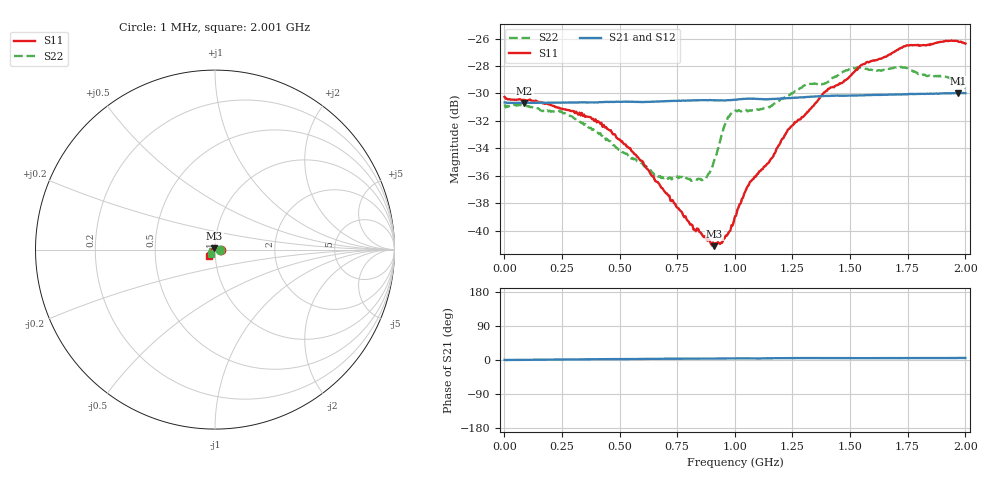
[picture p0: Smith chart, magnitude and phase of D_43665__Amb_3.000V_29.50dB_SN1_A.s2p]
! device id: 43665_
! dir: \\malibu\benchdata\1_engineers\tn_data\43665_75ohm\new\sparar\43665_\amb\3p000v\29p50db
! Serial: 1
! Insertion: A
! Temp: Amb
! VDD: 3.000V
! Attenuation Step: 29.50dB
! IDD: 1.450117e+00mA
! FILE NAME
! DATE 03-27-2009 08:40:42
! CORRECTED  DATA
#  Hz  S  RI  R  75
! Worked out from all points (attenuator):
!   401 points, 1 MHz to 2.001 GHz, reference 75 ohm
!   highest |S21| = -29.97 dB at 1.971 GHz (marker M1); lowest = -30.7 dB at 86 MHz (marker M2)
!   lowest |S11| = -41.1 dB at 911 MHz (marker M3), VSWR 1.02, Z = 74.4 + j1.16 ohm
!   |S11| at or under -10 dB: start of sweep to end of sweep
!   |S22| runs from -36.4 to -28.1 dB; largest |S21 - S12| = 0.00043
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1000000  0.0307 -0.000332  0.0293 0.000221  0.0293 -0.000151  0.0288 -0.000389
8.6e7  0.0299 0.00228  0.0292 0.000245  0.0292 0.000214  0.0283 0.0047
2.41e8  0.0272 0.00616  0.0293 0.000641  0.0293 0.000677  0.0245 0.0117
3.36e8  0.0256 0.00816  0.0293 0.000856  0.0293 0.000866  0.0195 0.0151
4.71e8  0.0197 0.0107  0.0294 0.0012  0.0295 0.00124  0.0118 0.0168
5.91e8  0.014 0.0113  0.0294 0.00139  0.0294 0.00141  0.0033 0.0174
6.71e8  0.00998 0.011  0.0295 0.00168  0.0295 0.00169  -0.00116 0.0157
8.66e8  -0.000993 0.00942  0.0298 0.00188  0.0298 0.00198  -0.0137 0.00713
9.11e8  -0.00409 0.00778  0.0298 0.00192  0.0298 0.00203  -0.0177 0.00389
9.61e8  -0.00677 0.00682  0.0298 0.00213  0.0298 0.0022  -0.0245 0.00322
1.001e9  -0.00933 0.00634  0.0299 0.00234  0.0299 0.0024  -0.027 0.00448
1.066e9  -0.0144 0.00441  0.0302 0.00226  0.0302 0.00234  -0.0274 0.00137
1.156e9  -0.0182 0.00122  0.0301 0.00245  0.0301 0.00256  -0.0283 -0.0028
1.236e9  -0.0234 -0.00229  0.0303 0.00262  0.0304 0.00277  -0.0302 -0.008
1.336e9  -0.0274 -0.00715  0.0307 0.00274  0.0307 0.00283  -0.0317 -0.013
1.396e9  -0.0304 -0.0108  0.0309 0.00265  0.0309 0.0028  -0.0302 -0.0167
1.471e9  -0.0317 -0.0144  0.0309 0.00262  0.031 0.00273  -0.0324 -0.0199
1.546e9  -0.0354 -0.0185  0.031 0.00268  0.0311 0.00271  -0.032 -0.0229
1.671e9  -0.0364 -0.0245  0.0312 0.00269  0.0313 0.0028  -0.03 -0.0247
1.756e9  -0.0367 -0.0298  0.0314 0.00276  0.0315 0.00277  -0.0274 -0.0273
1.971e9  -0.0333 -0.0357  0.0316 0.0029  0.0317 0.00257  -0.0228 -0.0264
2.001e9  -0.0321 -0.0358  0.0316 0.00294  0.0317 0.00255  -0.0213 -0.0252
